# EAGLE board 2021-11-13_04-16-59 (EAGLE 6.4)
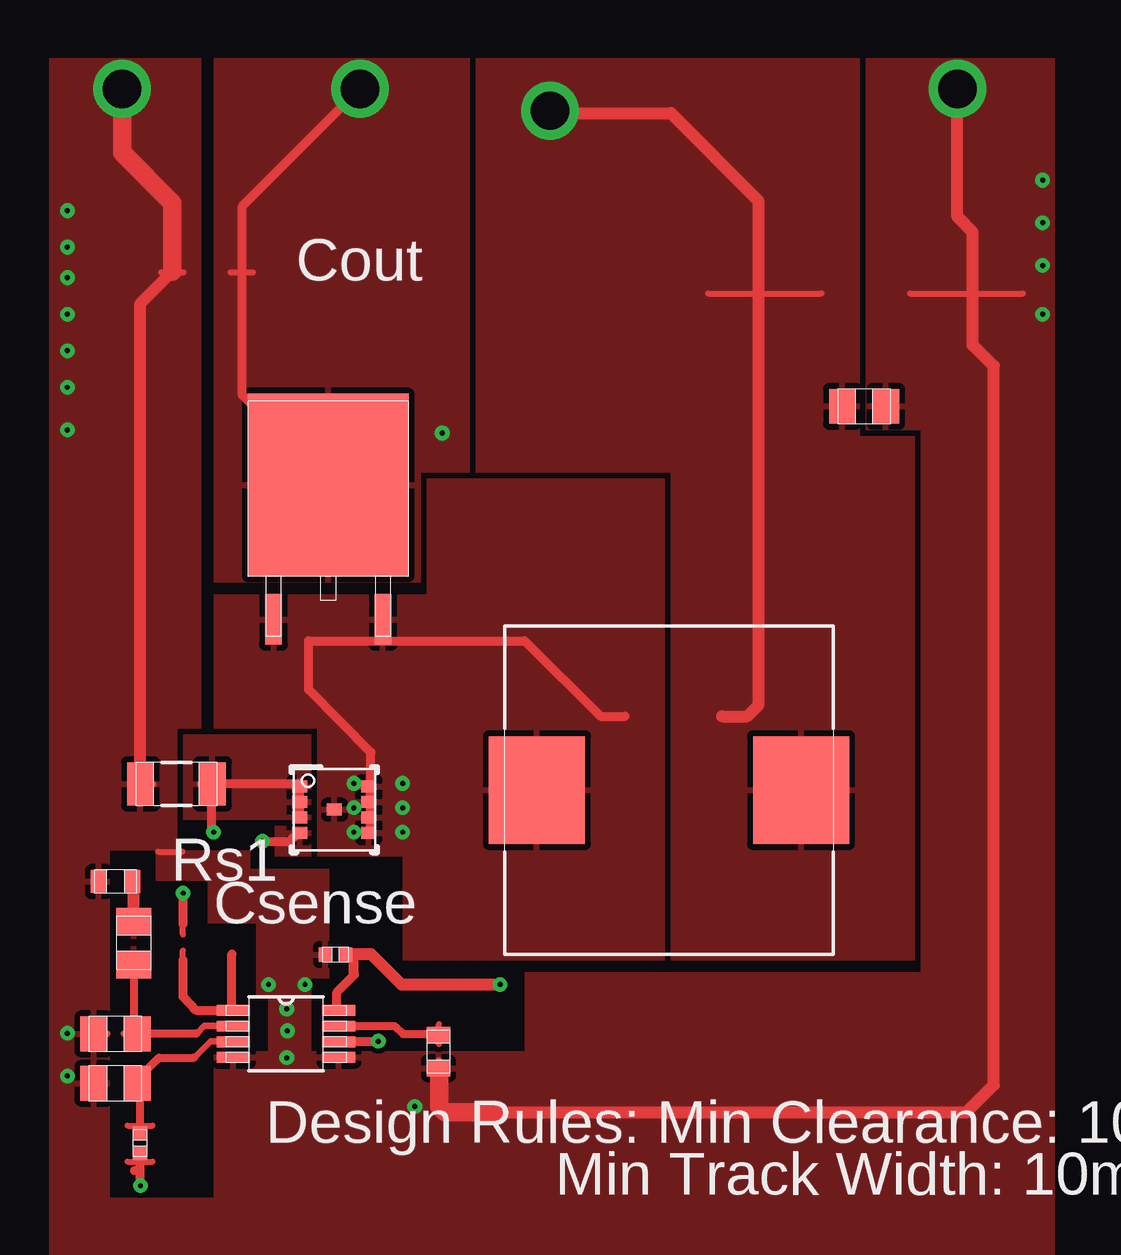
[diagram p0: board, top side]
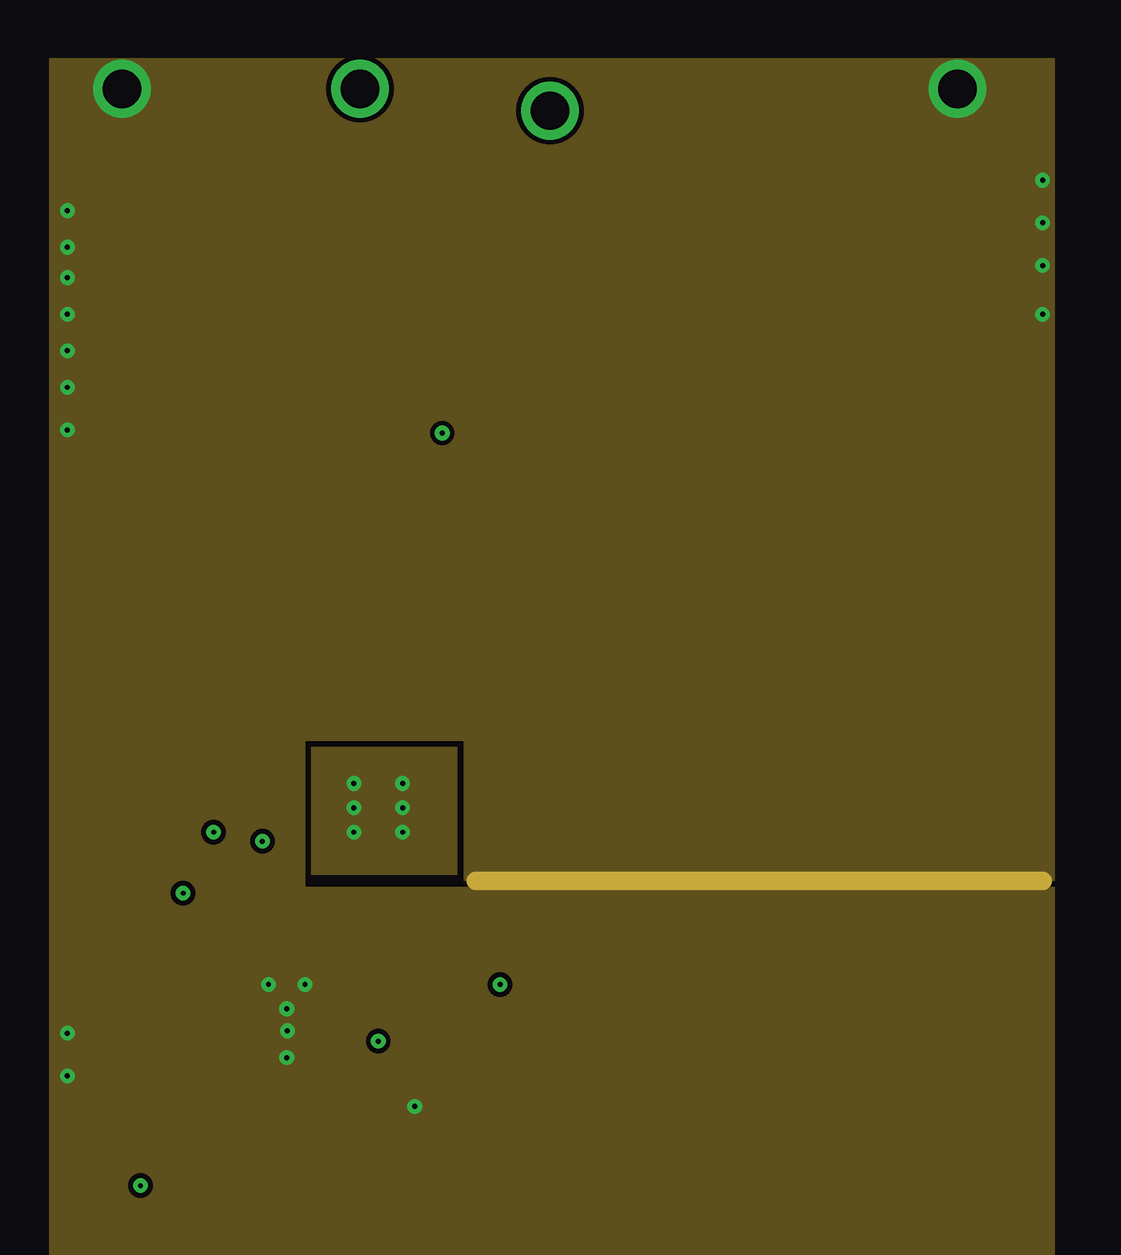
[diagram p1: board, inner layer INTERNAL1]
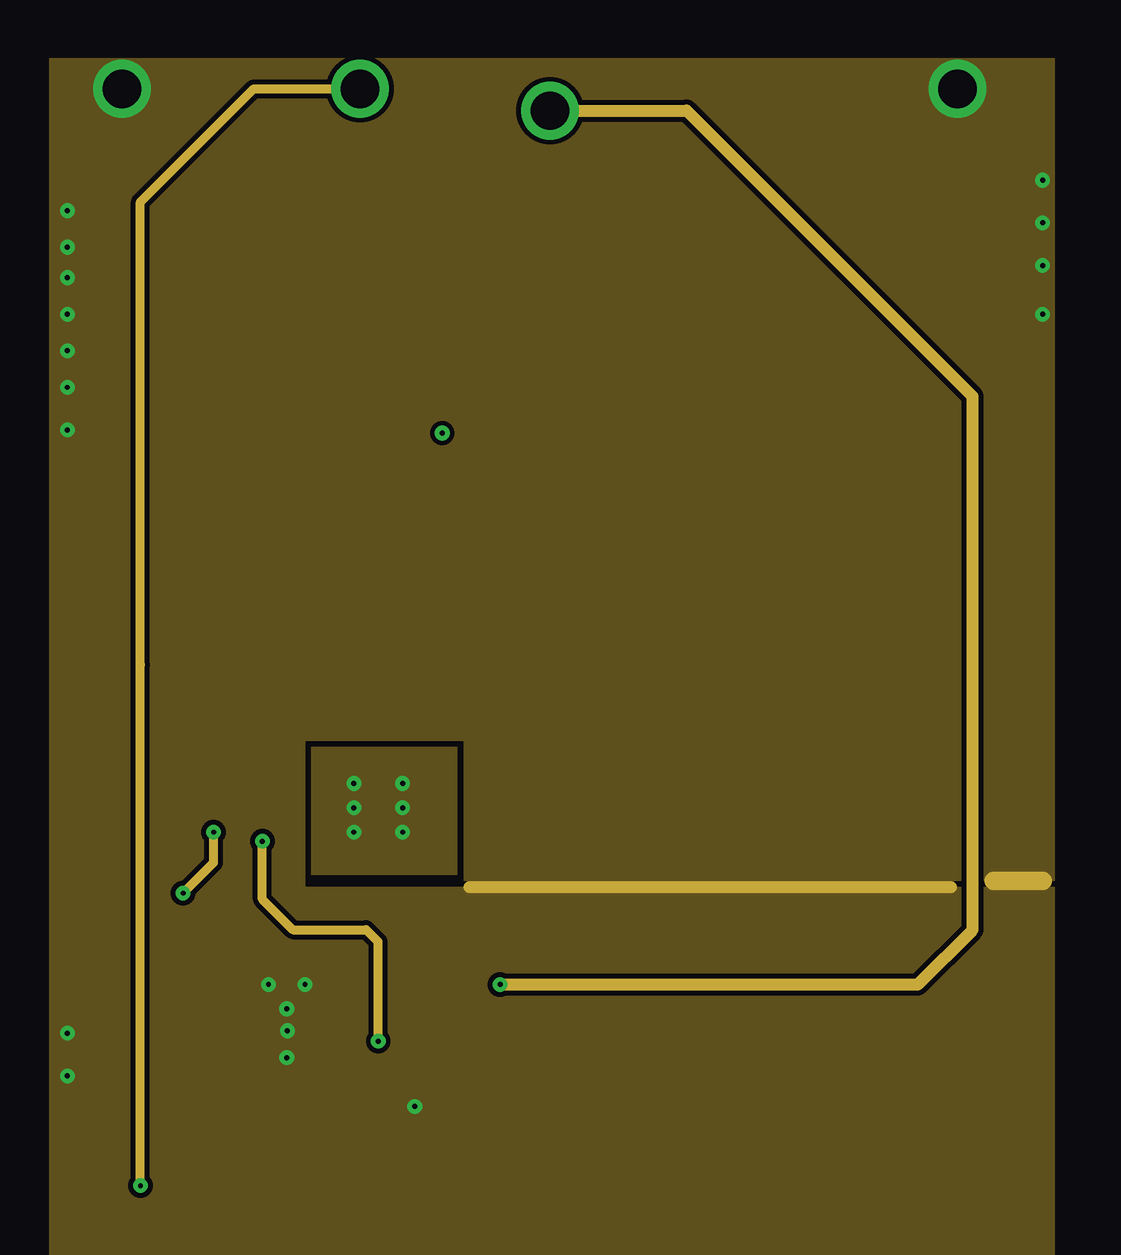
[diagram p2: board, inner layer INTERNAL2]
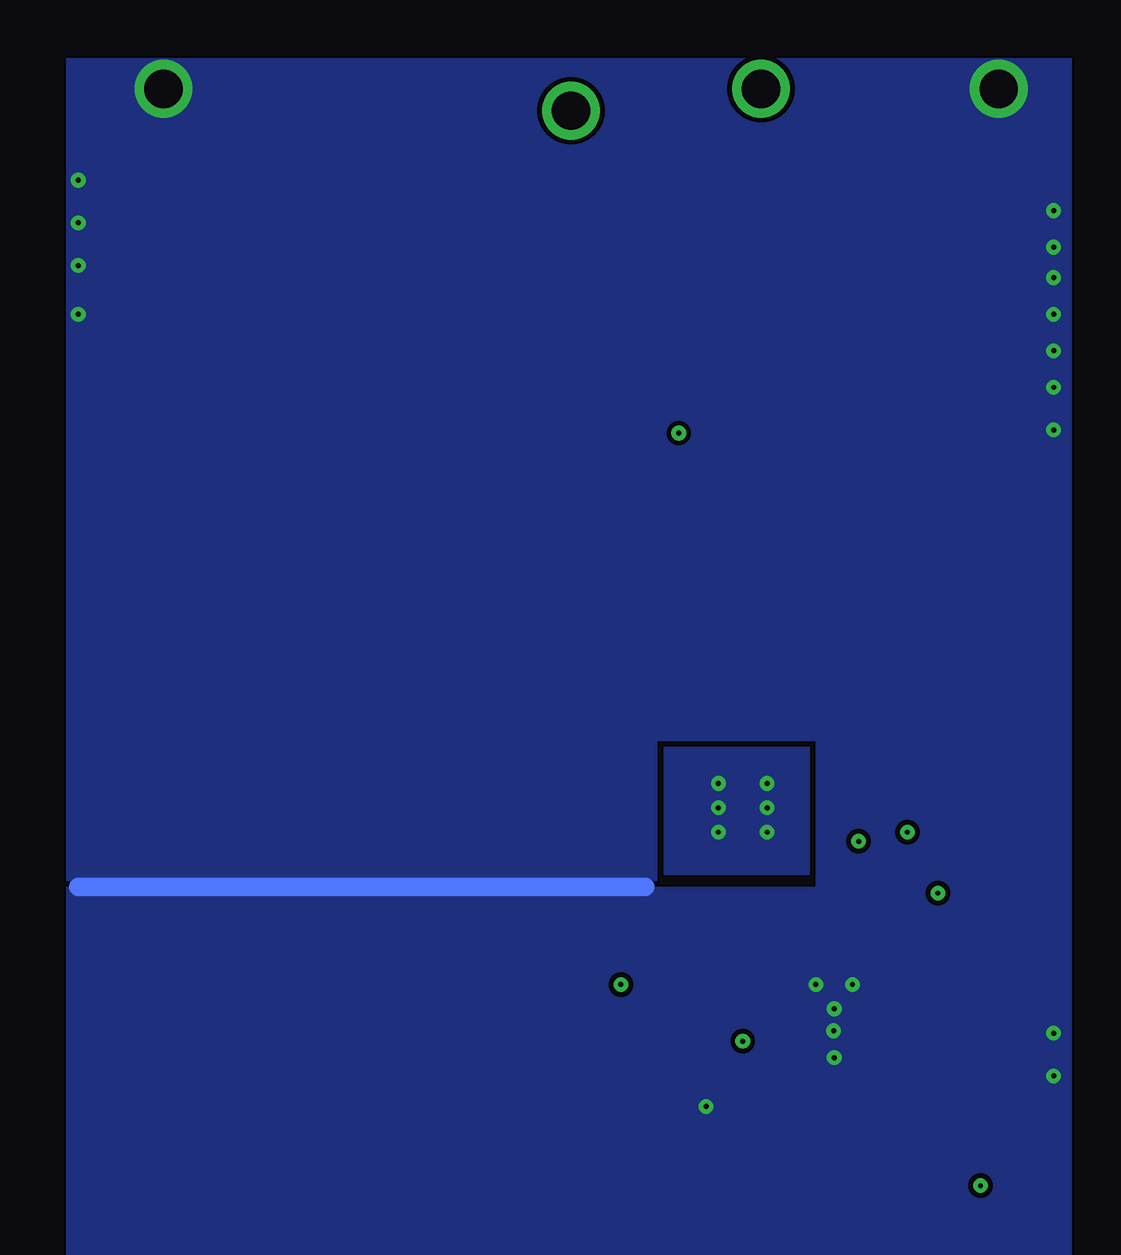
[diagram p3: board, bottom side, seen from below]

No outline drawn. Coordinates in mm, seen from the top.
Copper layers ((1*2)+(15*16)): TOP / INTERNAL1 / layer 15 / BOTTOM

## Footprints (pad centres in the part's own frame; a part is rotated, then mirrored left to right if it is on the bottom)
0402 = smd 0.559 x 0.61: 1 -0.419,0; 2 0.419,0
0805 = smd 1.118 x 1.448: 1 -0.902,0; 2 0.902,0
DPAK = smd 0.701 x 2.111: 1 -2.28,-5.45; 3 2.28,-5.45 | smd 6.7 x 7.605: 2 0,0.152
TP-1502 = drill 0.813 pad 1.651 round: 1 0,0
SRP1270 = smd 4 x 4.496: 1 -5.505,0; 2 5.505,0
DQG0008A = smd 0.63 x 0.5: 1 -1.435,0.975; 2 -1.435,0.325; 3 -1.435,-0.325; 4 -1.435,-0.975; 5 1.435,-0.975; 6 1.435,-0.325; 7 1.435,0.325; 8 1.435,0.975; 9 0,0
0603 = smd 0.66 x 0.965: 1 -0.699,0; 2 0.699,0
1206 = smd 1.118 x 1.803: 1 -1.499,0; 2 1.499,0
MUA08A = smd 1.372 x 0.457: 1 -2.197,0.975; 2 -2.197,0.325; 3 -2.197,-0.325; 4 -2.197,-0.975; 5 2.197,-0.975; 6 2.197,-0.325; 7 2.197,0.325; 8 2.197,0.975

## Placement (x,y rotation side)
Cbyp  [0402]  37.85,38.84 180 top
Ccomp  [0805]  29.44,39.32 90 top
Ccomp2  [0805]  28.68,35.53 180 top
Cin  [0805]  59.87,61.7 0 top
D1  [DPAK]  37.54,58.27 0 top
GND  [TP-1502]  63.73,74.88 0 top
GND1  [TP-1502]  28.93,74.88 180 top
L1  [SRP1270]  51.74,45.69 180 top
M1  [DQG0008A]  37.8,44.88 0 top
Rcomp  [0603]  28.68,41.88 180 top
Rfadj  [0603]  42.14,34.8 90 top
Rfb1  [0805]  28.68,33.48 180 top
Rfb2  [0402]  29.69,30.99 90 top
Rsense  [1206]  31.22,45.95 0 top
U1  [MUA08A]  35.79,35.53 0 top
VIN  [TP-1502]  46.79,73.99 0 top
VOUT  [TP-1502]  38.84,74.88 0 top

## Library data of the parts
Cbyp = ultra-librarian; RefDes: Cbyp; Type: GRM155R70J104KA01D
Ccomp = ultra-librarian; RefDes: Ccomp; Type: C0805C473J3GACTU
Ccomp2 = ultra-librarian; RefDes: Ccomp2; Type: C2012C0G1H272J060AA
Cin = ultra-librarian; RefDes: Cin; Type: C0805C106K8PACTU
D1 = ultra-librarian; RefDes: D1; Type: SBRD10200TR
GND = ultra-librarian; RefDes: GND; Type: TP-1502
GND1 VOUT = ultra-librarian
L1 = ultra-librarian; RefDes: L1; Type: SRP1270-3R3M
M1 = ultra-librarian; RefDes: M1; Type: CSD16327Q3
Rcomp = ultra-librarian; RefDes: Rcomp; Type: RC0603FR-072K2L
Rfadj = ultra-librarian; RefDes: Rfadj; Type: RC0603FR-0727KL
Rfb1 = ultra-librarian; RefDes: Rfb1; Type: RT0805BRD07101RL
Rfb2 = ultra-librarian; RefDes: Rfb2; Type: CRCW04021K50FKED
Rsense = ultra-librarian; RefDes: Rsense; Type: WSLP1206R0100FEA
U1 = ultra-librarian; RefDes: U1; Type: LM3478MM/NOPB
VIN = ultra-librarian; RefDes: VIN; Type: TP-1502

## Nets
0: Cbyp.2 Ccomp2.2 Cin.2 GND1.1 GND.1 Rcomp.2 Rfadj.1 Rfb1.2 Rsense.1 U1.4 U1.5
1: Cbyp.1 Cin.1 L1.1 U1.8 VIN.1
2: M1.1 M1.2 M1.3 Rsense.2
3: U1.1
4: Ccomp2.1 Ccomp.1 U1.2
5: D1.2 Rfb2.1 VOUT.1
6: D1.1 D1.3 L1.2 M1.5 M1.6 M1.7 M1.8 M1.9
7: Rfb1.1 Rfb2.2 U1.3
8: Ccomp.2 Rcomp.1
9: Rfadj.2 U1.7
10: M1.4 U1.6

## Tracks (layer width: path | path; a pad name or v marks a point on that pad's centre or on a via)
0  (via drill 0.2 pad 0.56, 1.6 pad 2.21)
  TOP 0.254: 30.45,43.13 31.47,43.13 | 29.31,45.95 30.25,45.95 | 42.15,33.6 42.15,34.44 | 27.93,32.99 27.93,34.04 | 27.51,35.55 28.35,35.55 | 61.77,66.4 66.5,66.4 | 30.58,67.28 31.52,67.28
  TOP 0.508: 31.04,67.31 29.72,65.96 29.72,46.02 29.77,45.97 | 63.75,74.3 63.75,69.6 64.39,68.94 64.39,66.42 64.39,64.24 65.28,63.37 65.28,33.4 64.14,32.26 44.45,32.26
  TOP 0.762: v28.96,74.93 28.96,72.26 31.04,70.16 31.04,67.31 | 42.16,34.04 42.16,32.51 42.42,32.26 44.45,32.26
  INTERNAL1 0.762: 43.69,41.91 67.31,41.91
  INTERNAL2 0.508: 43.43,41.66 63.5,41.66
  INTERNAL2 0.762: 65.28,41.91 67.31,41.91
  BOTTOM 0.762: 43.69,41.66 67.31,41.66
  other vias: 35.84,35.66 67.31,65.53 67.31,67.56 26.67,69.85 26.67,65.53 67.31,71.12 67.31,69.34 26.67,68.33 26.67,67.06 26.67,64.01 26.67,62.48 26.67,60.71 36.58,37.59 26.67,35.56 26.67,33.78 35.05,37.59 35.81,36.58 35.81,34.54 41.15,32.51 63.75,74.93
  pour TOP (rank 6): 59.94,76.2 67.82,76.2 67.82,25.91 25.91,25.91 25.91,76.2 32.26,76.2 32.26,48.26 31.24,48.26 31.24,43.18 28.45,43.18 28.45,28.7 32.77,28.7 32.77,34.8 35.05,34.8 35.05,37.08 34.54,37.08 34.54,40.13 32.51,40.13 32.51,41.91 30.35,41.91 30.35,43.05 31.37,43.18 34.29,43.18 34.29,42.42 37.59,42.42 37.59,37.85 36.83,37.85 36.83,34.8 45.72,34.8 45.72,38.1 62.23,38.1 62.23,60.71 59.94,60.71
  pour BOTTOM (rank 5): 25.91,76.2 25.91,25.91 67.82,25.91 67.82,41.66 36.58,41.66 36.58,47.75 43.18,47.75 43.18,41.91 67.82,41.91 67.82,76.2
  pour INTERNAL2 (rank 5): 25.91,76.2 25.91,25.91 67.82,25.91 67.82,41.66 36.58,41.66 36.58,47.75 43.18,47.75 43.18,41.91 67.82,41.91 67.82,76.2
  pour INTERNAL1 (rank 6): 25.91,76.2 25.91,25.91 67.82,25.91 67.82,41.66 36.58,41.66 36.58,47.75 43.18,47.75 43.18,41.91 67.82,41.91 67.82,76.2
1  (via drill 0.2 pad 0.56, 1.6 pad 2.21)
  TOP 0.254: 53.37,66.4 58.09,66.4
  TOP 0.381: 37.9,36.52 37.9,37.26 38.58,37.95 38.58,38.86 | 38.63,38 38.63,38.86
  TOP 0.508: 46.79,73.91 51.82,73.91 55.47,70.23 55.47,66.42 55.47,49.25 54.99,48.77 53.95,48.77 | v44.7,37.59 40.59,37.59 39.32,38.86 38.63,38.86 38.58,38.86
  INTERNAL2 0.508: v46.79,74.02 52.48,74.02 64.39,62.1 64.39,39.88 62.1,37.59 v44.7,37.59
  pour TOP (rank 2): 37.29,36.3 37.29,36.73 38.3,36.73 38.3,36.3
  pour TOP (rank 4): 51.82,38.61 61.98,38.61 61.98,60.45 59.69,60.45 59.69,76.2 43.69,76.2 43.69,58.93 51.82,58.93
2  (via drill 0.2 pad 0.56)
  TOP 0.254: 32.21,45.95 33.15,45.95 | 31.48,39.67 31.48,40.51
  TOP 0.381: v32.77,43.94 32.69,43.99 32.69,45.97 36.3,45.97 36.35,45.92 36.35,45.26 36.35,44.63 | 31.5,40.11 | 31.5,40.11 v31.5,41.4
  INTERNAL2 0.381: v31.5,41.4 32.77,42.67 v32.77,43.94
  pour TOP: 36.04,44.37 36.04,44.86 36.65,44.86 36.65,44.37
  pour TOP (rank 4): 36.83,44.45 31.5,44.45 31.5,48.01 36.83,48.01
3
  TOP 0.254: 31.48,38.18 31.48,39.01
  TOP 0.381: 33.53,38.86 33.53,36.7 33.71,36.52 32.03,36.52 31.5,37.08 31.5,38.61
  pour TOP (rank 2): 33.07,36.3 33.07,36.73 34.09,36.73 34.09,36.3
4
  TOP 0.254: 29.01,35.55 29.84,35.55
  TOP 0.279: 32.08,35.56 32.38,35.87 33.71,35.87
  TOP 0.33: 32.08,35.56 | 29.46,35.56 | 29.46,35.56 32.08,35.56 | 29.46,35.56 29.46,38.61
  pour TOP (rank 2): 33.07,35.64 33.07,36.07 34.09,36.07 34.09,35.64
  pour TOP (rank 3): 28.75,38 28.75,39.19 30.15,39.19 30.15,38
5  (via drill 0.2 pad 0.56, 1.6 pad 2.21)
  TOP 0.254: 29.18,30.21 30.23,30.21 | 33.48,67.28 34.42,67.28
  TOP 0.381: v38.86,74.93 33.96,70.03 33.96,67.31 33.96,62.15 37.85,58.29 37.85,57.84 | v29.72,29.21 29.72,30.23 | v29.72,29.21 | 29.46,29.84
  INTERNAL2 0.381: v29.72,29.21 29.72,50.93 29.72,70.21 34.44,74.93 v38.86,74.93
  other vias: 42.29,60.58
  pour TOP (rank 5): 32.77,76.2 43.43,76.2 43.43,58.93 41.4,58.93 41.4,54.36 32.77,54.36
6  (via drill 0.2 pad 0.56)
  TOP 0.381: 39.32,43.97 39.32,44.63 39.32,45.26 39.32,45.92 39.32,47.27 36.73,49.89 36.73,51.92 45.72,51.92 48.9,48.77 49.91,48.77
  other vias: 38.61,45.97 40.64,45.97 38.61,44.96 38.61,43.94 40.64,43.94 40.64,44.96
  pour TOP (rank 5): 37.08,42.93 40.64,42.93 40.64,38.61 51.56,38.61 51.56,58.67 41.66,58.67 41.66,53.85 32.77,53.85 32.77,48.26 37.08,48.26
  pour BOTTOM (rank 3): 36.83,47.5 36.83,42.16 42.93,42.16 42.93,47.5
  pour INTERNAL2 (rank 3): 36.83,47.5 36.83,42.16 42.93,42.16 42.93,47.5
  pour INTERNAL1 (rank 4): 36.83,47.5 42.93,47.5 42.93,42.16 36.83,42.16
7
  TOP 0.254: 29.18,31.71 30.23,31.71 | 29.43,32.99 29.43,34.04
  TOP 0.279: 33.71,35.23 32.64,35.23 31.95,34.54
  TOP 0.33: 31.95,34.54 30.48,34.54 29.46,33.53 29.44,33.53 29.72,33.25 29.72,31.73
  pour TOP (rank 2): 33.07,35 33.07,35.43 34.09,35.43 34.09,35
8
  TOP 0.508: 29.46,40.11 29.44,40.13 29.44,41.91
  pour TOP (rank 3): 28.75,39.5 28.75,40.69 30.15,40.69 30.15,39.5
9
  TOP 0.254: 42.15,35.1 42.15,35.94
  TOP 0.33: 37.9,35.87 40.31,35.87 40.66,35.53 42.16,35.53
  pour TOP: 37.29,35.64 37.29,36.07 38.3,36.07 38.3,35.64
10  (via drill 0.2 pad 0.56)
  TOP 0.381: 36.35,43.97 35.92,43.56 v34.8,43.56 | 37.9,35.23 39.6,35.23 v39.62,35.23
  INTERNAL2 0.381: v39.62,35.23 39.62,39.37 39.12,39.88 36.07,39.88 34.8,41.15 v34.8,43.56
  pour TOP: 36.04,43.71 36.04,44.2 36.65,44.2 36.65,43.71
  pour TOP: 37.29,35 37.29,35.43 38.3,35.43 38.3,35
  pour TOP (rank 4): 36.83,44.2 35.31,44.2 35.31,42.93 36.83,42.93

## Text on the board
ASSYNOTES: Cout | Rs1 | Csense | Design Rules: Min Clearance: 10mil | Min Track Width: 10mil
